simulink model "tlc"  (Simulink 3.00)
settings: Solver=ode45  SolverMode=SingleTasking  StartTime=0.0  StopTime=10000  RelTol=1e-3  AbsTol=1e-6
undefined symbols (not defined in the file or in its folder): Manual

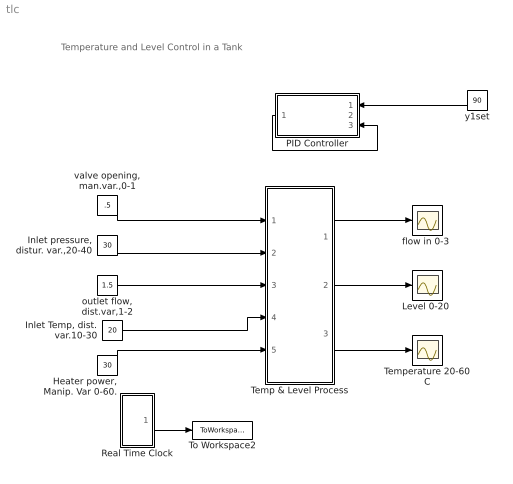
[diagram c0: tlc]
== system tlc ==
  note: Temperature and Level Control in a Tank
  "Heater power, Manip. Var 0-60." : Constant  Value=30
  "Inlet Temp, dist. var.10-30" : Constant  Value=20
  "Inlet pressure, distur. var.,20-40" : Constant  Value=30
  "Level 0-20 " : Scope
  PID Controller : Subsystem  Orientation=left  mask(Real PID Controller){am_flag=Manual, co=60, Ts=1, Kc=3.06, taui=64.4, taud=6.6, co_max=110, co_min=10, al=3}
      mask prompts: am_flag "Auto/Manual Switch"; co "Manual Controller Output"; Ts "Sample Time,Ts"; Kc "Kc: Proportional Gain: Negative for DIRECT Action"; taui "taui: Integral time"; taud "Derivative Time, taud"; co_max "Upper limit for controller output"; co_min "Lower limit for controller output"; al "Noise filter tim const, al"
      mask help: Programmed by Babu Joseph, Washington Universtiy in St. Louis, 1998
  Real Time Clock : Subsystem  mask(Sample time){Ts=1}
      mask prompts: Ts "Sample time"
      mask help: This block is used to set the sample time.
  Temp & Level Process : Subsystem  mask(Temperature and Level Control){finit=1.5, tinit=40, A=10, Ts=1, hinit=10}
      mask prompts: finit "Initial inlet flow"; tinit "Initial Temp in Tank"; A "Area"; Ts "Sample Time for PID controller"; hinit "Initial level in Tank"
      mask help: This block simulates a heated tank with water flowing through it. It has two manipulated inputs, three disturbance inputs and three controlled variables.
  Temperature 20-60 C : Scope
  To Workspace2 : ToWorkspace  VariableName=t  SampleTime=1  SaveFormat=Matrix
  "flow in 0-3 " : Scope
  "outlet flow, dist.var,1-2" : Constant  Value=1.5
  "valve opening, man.var.,0-1" : Constant  Value=.5
  y1set : Constant  Orientation=left  Value=90
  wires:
  Real Time Clock/1("Clock ") -> To Workspace2/1
  "valve opening, man.var.,0-1"/1 -> Temp & Level Process/1(xw)
  "Inlet pressure, distur. var.,20-40"/1 -> Temp & Level Process/2(ps)
  "outlet flow, dist.var,1-2"/1 -> Temp & Level Process/3(fout)
  Temp & Level Process/3(T) -> Temperature 20-60 C/1
  "Inlet Temp, dist. var.10-30"/1 -> Temp & Level Process/4(Tin)
  "Heater power, Manip. Var 0-60."/1 -> Temp & Level Process/5(Q)
  Temp & Level Process/1(fin) -> "flow in 0-3 "/1
  y1set/1 -> PID Controller/1(setpt)
  PID Controller/1(output) -> PID Controller/3(out_fdbk)
  Temp & Level Process/2(h) -> "Level 0-20 "/1

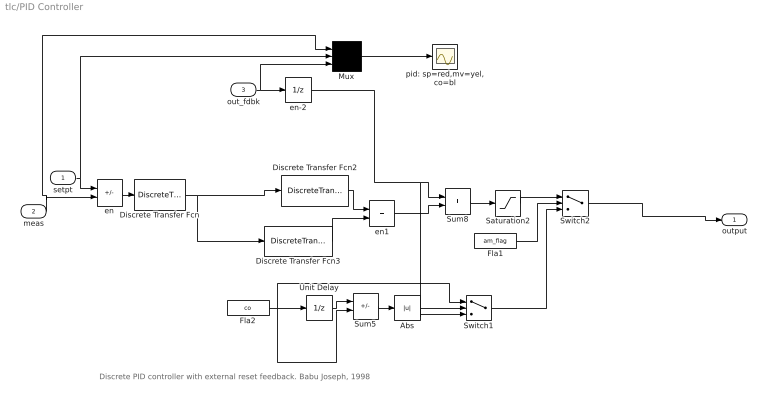
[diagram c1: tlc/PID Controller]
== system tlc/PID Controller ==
  note: Discrete PID controller with external reset feedback. Babu Joseph, 1998
  setpt : Inport  Port=1  PortWidth=-1  SampleTime=-1  DataType=auto
  meas : Inport  Port=2  PortWidth=-1  SampleTime=-1  DataType=auto
  out_fdbk : Inport  Port=3  PortWidth=-1  SampleTime=-1  DataType=auto
  Abs : Abs
  Discrete Transfer Fcn : DiscreteTransferFcn  Numerator="[Ts   0]"  Denominator="[(al+Ts)  -al]"  SampleTime=Ts
  Discrete Transfer Fcn2 : DiscreteTransferFcn  Numerator="Kc*[ (1+Ts/taui)  -1 ]"  Denominator="[ 1  0 ]"  SampleTime=Ts
  Discrete Transfer Fcn3 : DiscreteTransferFcn  Numerator=Kc*taud*[1 -2 1]  Denominator=[ 1 0 0]  SampleTime=Ts
  Fla1 : Constant  Value=am_flag
  Fla2 : Constant  Value=co
  Mux : Mux  Inputs=3
  Saturation2 : Saturate  UpperLimit=co_max  LowerLimit=co_min
  Sum5 : Sum  Inputs=+-  SaturateOnIntegerOverflow=on
  Sum8 : Sum  Inputs=++  SaturateOnIntegerOverflow=on
  Switch1 : Switch  Threshold=0.0001
  Switch2 : Switch  Threshold=1.5
  Unit Delay : UnitDelay  X0=0  SampleTime=Ts
  en : Sum  Inputs=+-  SaturateOnIntegerOverflow=on
  en-2 : UnitDelay  X0=co  SampleTime=Ts
  en1 : Sum  Inputs=++  SaturateOnIntegerOverflow=on
  pid: sp=red,mv=yel,co=bl : Scope
  output : Outport  Port=1  InitialOutput=0
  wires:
  Discrete Transfer Fcn/1 -> Discrete Transfer Fcn3/1, Discrete Transfer Fcn2/1
  en/1 -> Discrete Transfer Fcn/1
  setpt/1 -> Mux/2, en/1
  en1/1 -> Sum8/2
  Discrete Transfer Fcn2/1 -> en1/1
  Discrete Transfer Fcn3/1 -> en1/2
  Switch2/1 -> output/1
  en-2/1 -> Switch1/3, Sum8/1
  Switch1/1 -> Switch2/3
  Unit Delay/1 -> Sum5/1
  Fla2/1 -> Unit Delay/1, Sum5/2, Switch1/1
  Sum5/1 -> Abs/1
  Abs/1 -> Switch1/2
  Fla1/1 -> Switch2/2
  Saturation2/1 -> Switch2/1
  Sum8/1 -> Saturation2/1
  meas/1 -> en/2, Mux/1
  out_fdbk/1 -> en-2/1, Mux/3
  Mux/1 -> pid: sp=red,mv=yel,co=bl/1

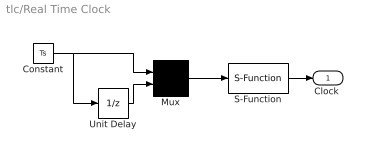
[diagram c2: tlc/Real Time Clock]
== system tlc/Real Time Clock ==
  Constant : Constant  Value=Ts
  Mux : Mux  Inputs=2
  S-Function : S-Function  FunctionName=wait3  PortCounts=[]  SFunctionModules=''
  Unit Delay : UnitDelay  X0=0  SampleTime=Ts
  "Clock " : Outport  Port=1  InitialOutput=0
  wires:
  S-Function/1 -> "Clock "/1
  Mux/1 -> S-Function/1
  Unit Delay/1 -> Mux/2
  Constant/1 -> Mux/1, Unit Delay/1

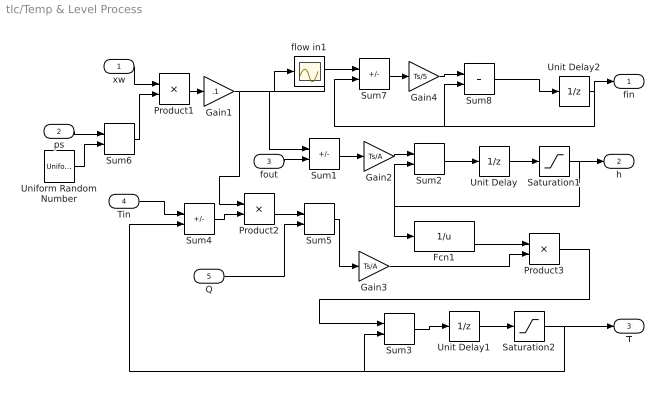
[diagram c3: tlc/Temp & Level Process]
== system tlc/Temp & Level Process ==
  xw : Inport  Port=1  PortWidth=-1  SampleTime=-1  DataType=auto
  ps : Inport  Port=2  PortWidth=-1  SampleTime=-1  DataType=auto
  fout : Inport  Port=3  PortWidth=-1  SampleTime=-1  DataType=auto
  Tin : Inport  Port=4  PortWidth=-1  SampleTime=-1  DataType=auto
  Q : Inport  Port=5  PortWidth=-1  SampleTime=-1  DataType=auto
  Fcn1 : Fcn  Expr=1/u
  Gain1 : Gain  Gain=.1  SaturateOnIntegerOverflow=on
  Gain2 : Gain  Gain=Ts/A  SaturateOnIntegerOverflow=on
  Gain3 : Gain  Gain=Ts/A  SaturateOnIntegerOverflow=on
  Gain4 : Gain  Gain=Ts/5  SaturateOnIntegerOverflow=on
  Product1 : Product  Inputs=2  SaturateOnIntegerOverflow=on
  Product2 : Product  Inputs=2  SaturateOnIntegerOverflow=on
  Product3 : Product  Inputs=2  SaturateOnIntegerOverflow=on
  Saturation1 : Saturate  UpperLimit=20  LowerLimit=1
  Saturation2 : Saturate  UpperLimit=60  LowerLimit=20
  Sum1 : Sum  Inputs=+-  SaturateOnIntegerOverflow=on
  Sum{2..3,5..6,8} (5 alike) : Sum  Inputs=++  SaturateOnIntegerOverflow=on
  Sum4 : Sum  Inputs=+-  SaturateOnIntegerOverflow=on
  Sum7 : Sum  Inputs=+-  SaturateOnIntegerOverflow=on
  Uniform Random Number : UniformRandomNumber  Minimum=-1  Maximum=1  Seed=0  SampleTime=1
  Unit Delay : UnitDelay  X0=hinit  SampleTime=Ts
  Unit Delay1 : UnitDelay  X0=tinit  SampleTime=Ts
  Unit Delay2 : UnitDelay  X0=finit  SampleTime=Ts
  flow in1 : Scope
  fin : Outport  Port=1  InitialOutput=0
  h : Outport  Port=2  InitialOutput=0
  T : Outport  Port=3  InitialOutput=0
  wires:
  Product1/1 -> Gain1/1
  Sum1/1 -> Gain2/1
  Gain2/1 -> Sum2/1
  Sum2/1 -> Unit Delay/1
  Unit Delay/1 -> Saturation1/1
  Saturation1/1 -> h/1, Sum2/2, Fcn1/1
  xw/1 -> Product1/1
  fout/1 -> Sum1/2
  Tin/1 -> Sum4/1
  Gain1/1 -> Sum1/1, Sum7/1, flow in1/1, Product2/1
  Sum4/1 -> Product2/2
  Product2/1 -> Sum5/1
  Q/1 -> Sum5/2
  Sum5/1 -> Gain3/1
  Sum3/1 -> Unit Delay1/1
  Unit Delay1/1 -> Saturation2/1
  Saturation2/1 -> T/1, Sum3/2, Sum4/2
  Fcn1/1 -> Product3/1
  Gain3/1 -> Product3/2
  Product3/1 -> Sum3/1
  ps/1 -> Sum6/1
  Uniform Random Number/1 -> Sum6/2
  Sum6/1 -> Product1/2
  Sum7/1 -> Gain4/1
  Gain4/1 -> Sum8/1
  Unit Delay2/1 -> fin/1, Sum7/2, Sum8/2
  Sum8/1 -> Unit Delay2/1
